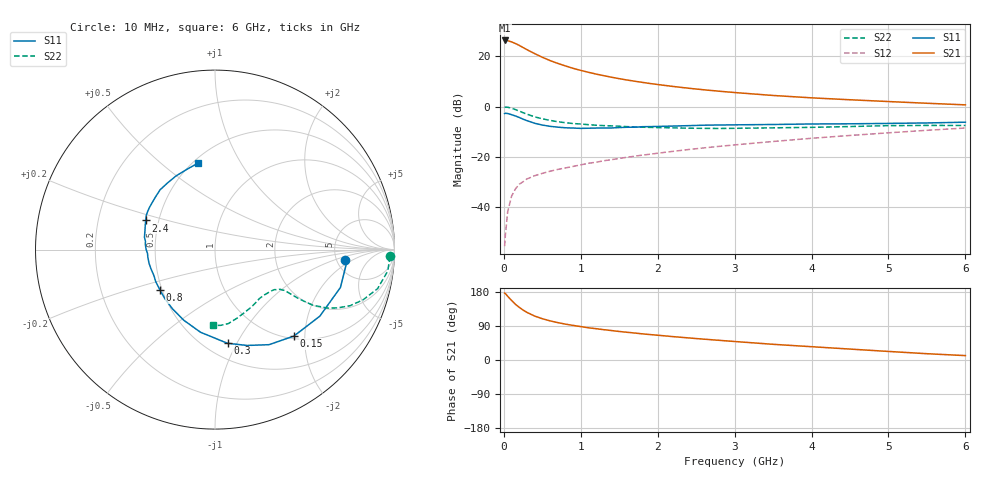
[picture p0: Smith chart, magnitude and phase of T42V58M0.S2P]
! Infineon Technologies  Discrete & RF Semiconductors
! BFR182T
! Si NPN RF Bipolar Junction Transistor in SC75
! VCE = 2.5 V  IC = 8 mA
! Common Emitter S-Parameters:  October  1999
# GHz  S  MA  R  50
!  f  S11  S21  S12  S22
! GHz  MAG  ANG  MAG  ANG  MAG  ANG  MAG  ANG
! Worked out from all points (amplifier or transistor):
!   36 points, 10 MHz to 6 GHz, reference 50 ohm
!   highest |S21| = 26.3 dB at 10 MHz (marker M1)
!   |S21| within 3 dB of that: start of sweep to 261.5 MHz
!   unconditionally stable (mu >= 1): 1.12 GHz to 3.846 GHz
!   at 250 MHz: K = 0.40, MSG = 26.6 dB, |S12| = -29.8 dB
!   at 1.4 GHz: K = 1.07, MAG = 14.8 dB, |S12| = -21.1 dB
!   at 6 GHz: K = 0.84, MSG = 4.6 dB, |S12| = -8.5 dB
!   lowest NFmin = 1.40 dB at 450 MHz
!   S11 on the Smith chart (normalised r, x): 10 MHz: 6.00, -1.50; 150 MHz: 1.05, -1.76; 300 MHz: 0.64, -0.92; 800 MHz: 0.49, -0.25; 2.4 GHz: 0.42, +0.17; 6 GHz: 0.53, +0.67
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0.01  0.729 -4.6  20.54 176.7  0.0017 83.3  0.9769 -2.2
0.02  0.7377 -5.3  20.52 175.5  0.0028 92.9  0.9752 -2.8
0.05  0.73 -16.8  20.31 168.1  0.0082 82.5  0.9697 -7.1
0.1  0.6919 -32.4  19.24 157.3  0.0166 76.5  0.9317 -13.5
0.15  0.6522 -47.6  17.89 147.2  0.0232 69.0  0.8717 -18.7
0.2  0.6093 -60.4  16.39 138.9  0.0288 66.2  0.8144 -22.6
0.25  0.5631 -71.5  14.87 131.8  0.0323 61.2  0.7569 -25.4
0.3  0.5266 -82.4  13.51 125.7  0.0366 59.0  0.7088 -27.4
0.4  0.4676 -99.9  11.27 116.0  0.0425 56.5  0.627 -29.6
0.5  0.4304 -113.8  9.539 109.0  0.0473 56.6  0.5727 -30.1
0.6  0.4064 -125.6  8.203 103.3  0.0521 56.9  0.5326 -30.4
0.7  0.3911 -135.5  7.206 98.7  0.0567 57.4  0.5018 -30.4
0.8  0.3801 -143.9  6.416 94.7  0.0606 57.5  0.4789 -30.4
1.1  0.3727 -163.6  4.794 85.0  0.0751 60.6  0.4382 -30.9
1.3  0.3763 -172.9  4.109 80.0  0.0842 61.8  0.4196 -31.9
1.6  0.3892 175.8  3.375 73.2  0.0988 63.2  0.4005 -33.8
2.2  0.411 161.0  2.512 61.7  0.1295 64.7  0.3787 -40.2
2.4  0.4188 157.2  2.317 58.3  0.1405 65.0  0.3728 -42.8
3.5  0.4416 139.3  1.663 41.4  0.2032 63.0  0.3788 -57.6
4.5  0.4557 125.8  1.367 28.8  0.2676 59.1  0.4021 -72.6
5.5  0.4739 109.3  1.165 16.6  0.3386 53.7  0.4232 -85.7
6  0.4904 101.3  1.083 11.6  0.3759 50.1  0.4225 -91.2
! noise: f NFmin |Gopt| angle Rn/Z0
0.45  1.4  0.26  41  0.29
0.9  1.5  0.25  83  0.23
1.8  2  0.21  162  0.2
